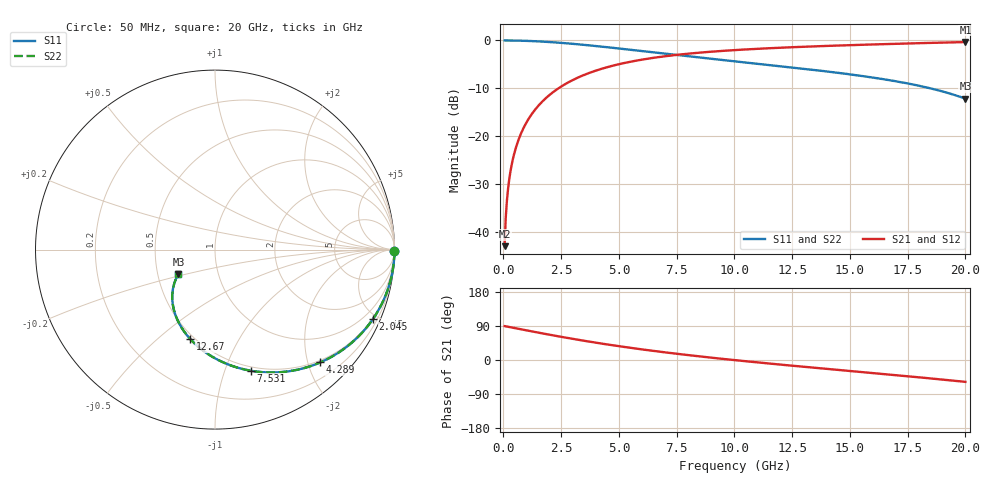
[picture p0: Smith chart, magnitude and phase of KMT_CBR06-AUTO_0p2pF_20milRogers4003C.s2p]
! Data measured by Modelithics Inc. support@modelithics.com 813-866-6335
! KEMET CBR06-AUTO 0.2pF, Pad Width= 0.851mm, Pad Length= 0.64mm, Pad Gap= 0.62mm, 20mil Rogers 4003C substrate Data, January 2022
# hz S ma R 50
! 2 Port Network Data from SP1.SP block
! freq  magS11  angS11  magS21  angS21  magS12  angS12  magS22  angS22
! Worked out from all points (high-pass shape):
!   401 points, 50 MHz to 20 GHz, reference 50 ohm
!   highest |S21| = -0.34 dB at 20 GHz (marker M1); lowest = -43.1 dB at 50 MHz (marker M2)
!   |S21| within 3 dB of the highest: 6.945 GHz to end of sweep
!   lowest |S11| = -12.2 dB at 20 GHz (marker M3), VSWR 1.65, Z = 32 - j9.33 ohm
!   |S11| at or under -10 dB: 18.47 GHz to end of sweep
!   |S22| runs from -12.2 to 0.0 dB; largest |S21 - S12| = 0
!   S11 on the Smith chart (normalised r, x): 50 MHz: open; 2.045 GHz: 0.46, -4.70; 4.289 GHz: 0.46, -2.22; 7.531 GHz: 0.46, -1.23; 12.67 GHz: 0.48, -0.64; 20 GHz: 0.64, -0.19
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5e7  1 -0.6  0.00703 89.4  0.00703 89.4  1 -0.6
9.9875e7  0.9999 -1.2  0.01404 88.8  0.01404 88.8  0.9999 -1.2
1.99625e8  0.9996 -2.4  0.02806 87.6  0.02806 87.6  0.9996 -2.4
2.99375e8  0.9991 -3.6  0.04205 86.4  0.04205 86.4  0.9991 -3.6
4.49e8  0.998 -5.3  0.06299 84.7  0.06299 84.7  0.998 -5.3
5.98625e8  0.9964 -7.1  0.08384 82.9  0.08384 82.9  0.9964 -7.1
8.48e8  0.9929 -10.0  0.1183 79.9  0.1183 79.9  0.9929 -10.0
1.197125e9  0.986 -14.1  0.1657 75.8  0.1657 75.8  0.986 -14.1
1.596125e9  0.9757 -18.7  0.2183 71.2  0.2183 71.2  0.9757 -18.7
2.045e9  0.9611 -23.8  0.275 66.2  0.275 66.2  0.9611 -23.8
2.6435e9  0.9378 -30.3  0.3458 59.6  0.3458 59.6  0.9378 -30.3
3.391625e9  0.9041 -38.2  0.4256 51.8  0.4256 51.8  0.9041 -38.2
4.289375e9  0.8599 -46.9  0.5084 43.0  0.5084 43.0  0.8599 -46.9
5.4365e9  0.8021 -57.2  0.5948 32.7  0.5948 32.7  0.8021 -57.2
6.73325e9  0.7395 -67.6  0.6704 22.2  0.6704 22.2  0.7395 -67.6
7.53125e9  0.7036 -73.6  0.7077 16.2  0.7077 16.2  0.7036 -73.6
1.0025e10  0.6047 -90.1  0.7931 -0.4  0.7931 -0.4  0.6047 -90.1
1.266838e10  0.516 -105.6  0.8529 -16.0  0.8529 -16.0  0.516 -105.6
1.336662e10  0.4939 -109.5  0.8657 -19.9  0.8657 -19.9  0.4939 -109.5
1.670825e10  0.384 -127.8  0.9186 -38.4  0.9186 -38.4  0.384 -127.8
1.850375e10  0.3146 -137.7  0.9433 -48.7  0.9433 -48.7  0.3146 -137.7
2e10  0.2457 -146.1  0.9618 -57.7  0.9618 -57.7  0.2457 -146.1
